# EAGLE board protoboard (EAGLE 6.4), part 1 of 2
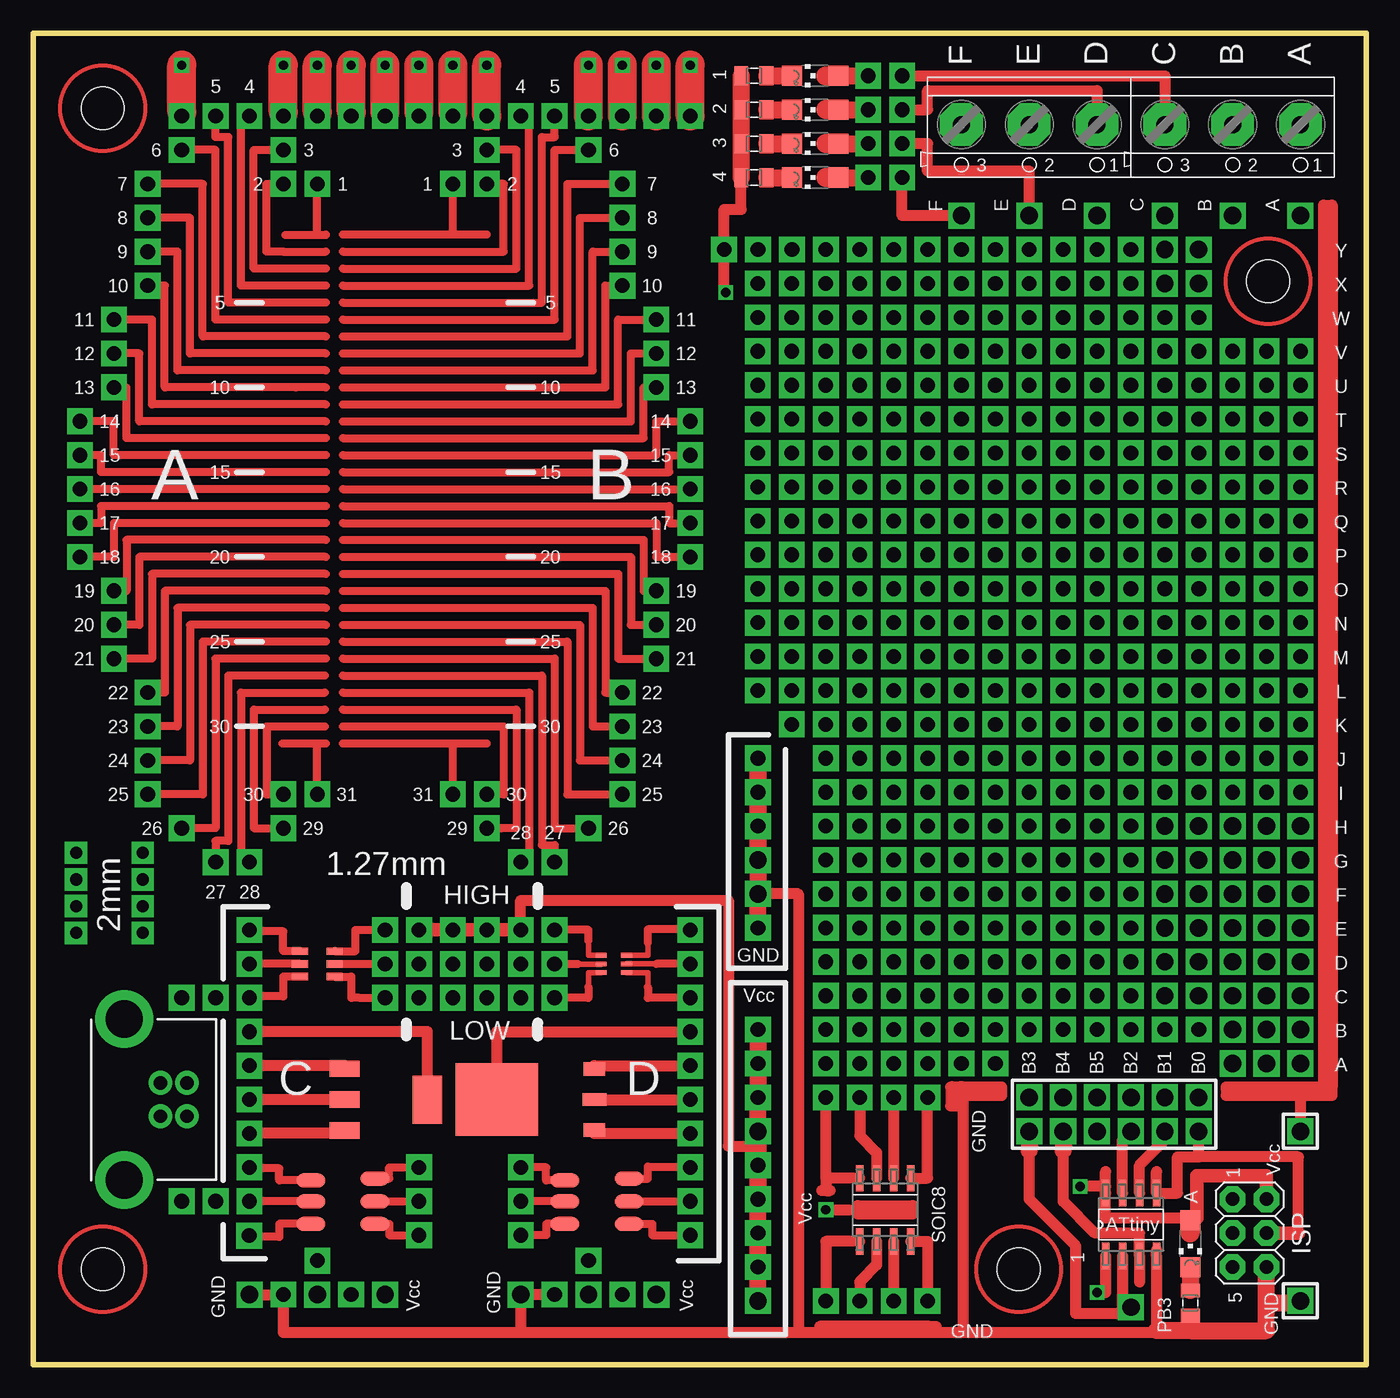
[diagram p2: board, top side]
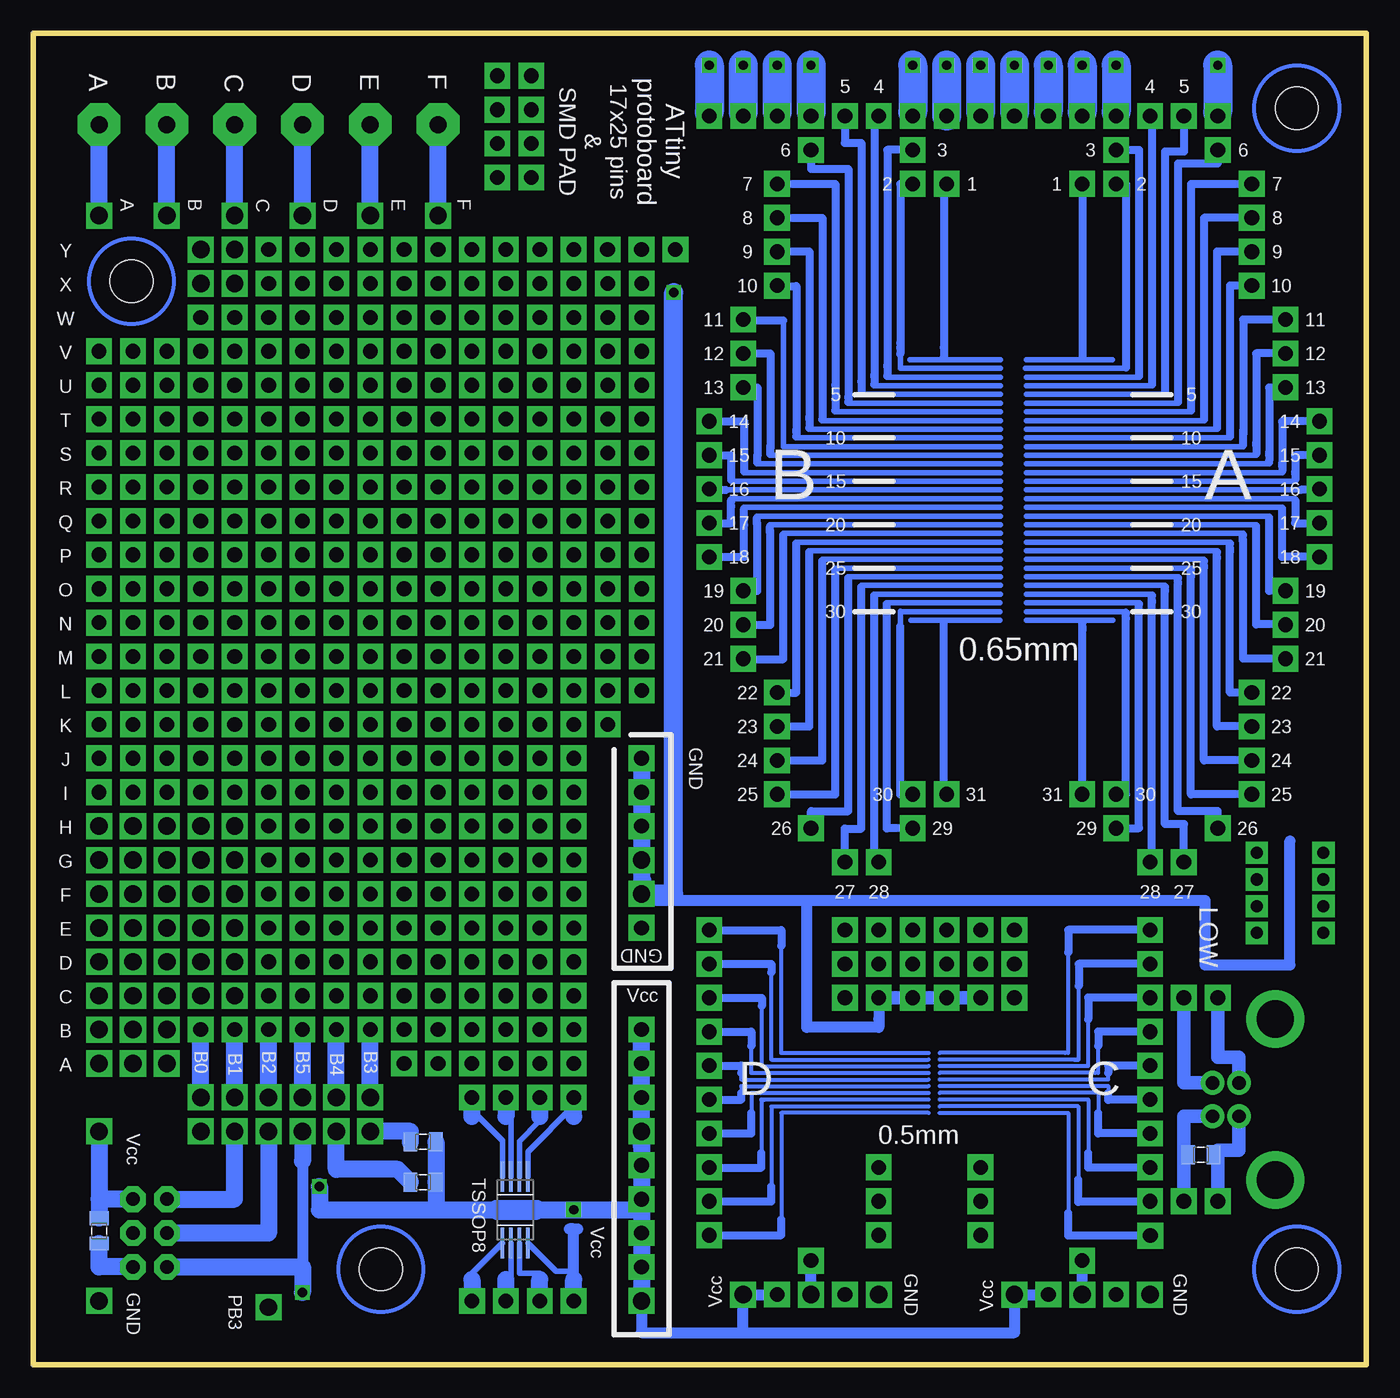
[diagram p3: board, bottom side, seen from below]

Size 99.85 x 99.7 mm. Coordinates in mm from the lower left corner, seen from the top.
Outline: 0,0 99.85,0 99.85,99.7 0,99.7 0,0
Copper layers (1*16): Top 0.035mm / dielectric 1.5mm / Bottom 0.035mm
Design rules "default *": minimum track width 10mil, minimum drill 24mil, track to track 7mil, track to pad 8mil, pad to pad 8mil, via to via 8mil, smd to smd 8mil, copper to edge 40mil, drill to drill 8mil, minimum pad ring 10mil, minimum via ring 8mil, stop-mask expansion 4mil, vias tented up to drill 0mil, thermal gap 10mil
Holes 3.2 mm at 73.82,7.14 5.19,7.14 5.19,94.08 92.51,81.12

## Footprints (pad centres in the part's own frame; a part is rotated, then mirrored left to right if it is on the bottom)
1X01 = drill 1.3 square: 1 0,0
SOIC127P600X175-8N = smd 1.981 x 0.559: 1 -2.362,1.905; 2 -2.362,0.635; 3 -2.362,-0.635; 4 -2.362,-1.905; 5 2.362,-1.905; 6 2.362,-0.635; 7 2.362,0.635; 8 2.362,1.905
0805 = smd 1.016 x 1.422: 1 -0.953,0; 2 0.953,0
TSSOP8 = smd 2.286 x 0.254: 1 -2.489,1.016; 2 -2.489,0.381; 3 -2.489,-0.254; 4 -2.489,-0.889; 5 2.489,-0.889; 6 2.489,-0.254; 7 2.489,0.381; 8 2.489,1.016
SC70-5 = smd 0.35 x 0.8: 1 -0.65,-0.95; 2 0,-0.95; 3 0.65,-0.95; 4 0.65,0.95; 5 -0.015,0.95; 6 -0.65,0.95
SOT23-5 = smd 0.55 x 1.2: 1 -0.95,-1.3; 2 0,-1.3; 3 0.95,-1.3; 4 0.95,1.3; 5 0,1.304; 6 -0.95,1.3
1X01' = drill 1.1 pad 1.93 square: 1 0,0
CZM_5/3 = drill 1.27 pad 3.2 octagon: 1 -5.08,0; 2 0,0; 3 5.08,0
CHIPLED_1206 = smd 1.5 x 1.5: A 0,-1.75; C 0,1.75
2X03 = drill 1.016 pad 1.93 octagon: 1 -2.54,-1.27; 2 -2.54,1.27; 3 0,-1.27; 4 0,1.27; 5 2.54,-1.27; 6 2.54,1.27
LED-TRICOLOR-5050-IC = smd 2.184 x 1.067: 1 -2.4,1.573; 2 -2.4,0; 3 -2.4,-1.7; 4 2.4,-1.7; 5 2.4,0; 6 2.4,1.7
SOT223 = smd 1.219 x 2.235: P-B 0,-3.099; P-C 2.311,-3.099; P_A -2.311,-3.099 | smd 3.6 x 2.2: P_POUZDRO 0,3.099
TO-252 = smd 1 x 1.6: P-A 2.28,-4.8; P-C -2.28,-4.8 | smd 0.914 x 1.778: P-B 0,-4.826 | smd 5.4 x 6.2: P_POUZDRO 0,2.5
USB-B-PTH = drill 1 pad 1.778: D+ 0,1.25; D- 1.981,1.25; GND 0,-1.25; VBUS 1.981,-1.25 | drill 2.8 pad 4.318: P$2 -2.718,6.02; SHIELD -2.718,-6.02

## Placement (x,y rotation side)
ARK-A  [1X01]  94.93,86.04 90 top
ARK-B  [1X01]  89.85,86.04 90 top
ARK-C  [1X01]  84.77,86.04 90 top
ARK-D  [1X01]  79.69,86.04 90 top
ARK-E  [1X01]  74.61,86.04 90 top
ARK-F  [1X01]  69.53,86.04 90 top
ATTINY  ATTINY__  [SOIC127P600X175-8N]  82.23,10.48 90 top
C1  [0805]  12.38,15.72 0 bottom
C8  1uF  [0805]  94.93,10 270 bottom
EMPTY1  SOIC-NIC  [SOIC127P600X175-8N]  63.82,11.59 90 top
EMPTY2  TSSOP-NIC  [TSSOP8]  63.82,11.59 270 bottom
IC1  AD8519KS  [SC70-5]  43.5,30 90 top
IC2  AD8519RJ  [SOT23-5]  21.27,30 90 top
J-A1  [1X01]  94.93,22.54 90 top
J-A2  [1X01]  92.39,22.54 90 top
J-A3  [1X01]  89.85,22.54 90 top
J-A10  [1X01']  72.07,22.54 90 top
J-A11  [1X01']  69.53,22.54 90 top
J-A12  [1X01']  66.99,22.54 90 top
J-A13  [1X01']  64.45,22.54 90 top
J-A14  [1X01']  61.91,22.54 90 top
J-A15  [1X01']  59.37,22.54 90 top
J-B1  [1X01]  94.93,25.08 90 top
J-B2  [1X01]  92.39,25.08 90 top
J-B3  [1X01]  89.85,25.08 90 top
J-B4  [1X01']  87.31,25.08 0 top
J-B5  [1X01']  84.77,25.08 0 top
J-B6  [1X01']  82.23,25.08 0 top
J-B7  [1X01']  79.69,25.08 0 top
J-B8  [1X01']  77.15,25.08 0 top
J-B9  [1X01']  74.61,25.08 0 top
J-B10  [1X01']  72.07,25.08 90 top
J-B11  [1X01']  69.53,25.08 90 top
J-B12  [1X01']  66.99,25.08 90 top
J-B13  [1X01']  64.45,25.08 90 top
J-B14  [1X01']  61.91,25.08 90 top
J-B15  [1X01']  59.37,25.08 90 top
J-C1  [1X01]  94.93,27.62 90 top
J-C2  [1X01]  92.39,27.62 90 top
J-C3  [1X01]  89.85,27.62 90 top
J-C4  [1X01]  87.31,27.62 90 top
J-C5  [1X01]  84.77,27.62 90 top
J-C6  [1X01']  82.23,27.62 90 top
J-C7  [1X01']  79.69,27.62 90 top
J-C8  [1X01']  77.15,27.62 90 top
J-C9  [1X01']  74.61,27.62 90 top
J-C10  [1X01']  72.07,27.62 90 top
J-C11  [1X01']  69.53,27.62 90 top
J-C12  [1X01']  66.99,27.62 90 top
J-C13  [1X01']  64.45,27.62 90 top
J-C14  [1X01']  61.91,27.62 90 top
J-C15  [1X01']  59.37,27.62 90 top
J-D1  [1X01]  94.93,30.16 90 top
J-D2  [1X01]  92.39,30.16 90 top
J-D3  [1X01]  89.85,30.16 90 top
J-D4  [1X01]  87.31,30.16 90 top
J-D5  [1X01]  84.77,30.16 90 top
J-D6  [1X01']  82.23,30.16 90 top
J-D7  [1X01']  79.69,30.16 90 top
J-D8  [1X01']  77.15,30.16 90 top
J-D9  [1X01']  74.61,30.16 90 top
J-D10  [1X01']  72.07,30.16 90 top
J-D11  [1X01']  69.53,30.16 90 top
J-D12  [1X01']  66.99,30.16 90 top
J-D13  [1X01']  64.45,30.16 90 top
J-D14  [1X01']  61.91,30.16 90 top
J-D15  [1X01']  59.37,30.16 90 top
J-E1  [1X01]  94.93,32.7 0 top
J-E2  [1X01]  92.39,32.7 0 top
J-E3  [1X01]  89.85,32.7 90 top
J-E4  [1X01]  87.31,32.7 90 top
J-E5  [1X01]  84.77,32.7 90 top
J-E6  [1X01']  82.23,32.7 90 top
J-E7  [1X01']  79.69,32.7 90 top
J-E8  [1X01']  77.15,32.7 90 top
J-E9  [1X01']  74.61,32.7 90 top
J-E10  [1X01']  72.07,32.7 90 top
J-E11  [1X01']  69.53,32.7 90 top
J-E12  [1X01']  66.99,32.7 0 top
J-E13  [1X01']  64.45,32.7 0 top
J-E14  [1X01']  61.91,32.7 0 top
J-E15  [1X01']  59.37,32.7 0 top
J-F1  [1X01]  94.93,35.24 0 top
J-F2  [1X01]  92.39,35.24 0 top
J-F3  [1X01]  89.85,35.24 0 top
J-F4  [1X01]  87.31,35.24 0 top
J-F5  [1X01]  84.77,35.24 0 top
J-F6  [1X01']  82.23,35.24 0 top
J-F7  [1X01']  79.69,35.24 0 top
J-F8  [1X01']  77.15,35.24 0 top
J-F9  [1X01']  74.61,35.24 0 top
J-F10  [1X01']  72.07,35.24 0 top
J-F11  [1X01']  69.53,35.24 90 top
J-F12  [1X01']  66.99,35.24 0 top
J-F13  [1X01']  64.45,35.24 0 top
J-F14  [1X01']  61.91,35.24 90 top
J-F15  [1X01']  59.37,35.24 90 top
J-G1  [1X01]  94.93,37.78 0 top
J-G2  [1X01]  92.39,37.78 0 top
J-G3  [1X01]  89.85,37.78 0 top
J-G4  [1X01]  87.31,37.78 0 top
J-G5  [1X01]  84.77,37.78 0 top
J-G6  [1X01']  82.23,37.78 0 top
J-G7  [1X01']  79.69,37.78 0 top
J-G8  [1X01']  77.15,37.78 0 top
J-G9  [1X01']  74.61,37.78 0 top
J-G10  [1X01']  72.07,37.78 0 top
J-G11  [1X01']  69.53,37.78 0 top
J-G12  [1X01']  66.99,37.78 0 top
J-G13  [1X01']  64.45,37.78 0 top
J-G14  [1X01']  61.91,37.78 0 top
J-G15  [1X01']  59.37,37.78 0 top
J-H1  [1X01]  94.93,40.32 0 top
J-H2  [1X01]  92.39,40.32 0 top
J-H3  [1X01]  89.85,40.32 0 top
J-H4  [1X01]  87.31,40.32 0 top
J-H5  [1X01]  84.77,40.32 0 top
J-H6  [1X01']  82.23,40.32 0 top
J-H7  [1X01']  79.69,40.32 0 top
J-H8  [1X01']  77.15,40.32 0 top
J-H9  [1X01']  74.61,40.32 0 top
J-H10  [1X01']  72.07,40.32 0 top
J-H11  [1X01']  69.53,40.32 0 top
J-H12  [1X01']  66.99,40.32 0 top
J-H13  [1X01']  64.45,40.32 0 top
J-H14  [1X01']  61.91,40.32 0 top
J-H15  [1X01']  59.37,40.32 0 top
J-HL-1  [1X01']  28.89,30 0 top
J-HL-2  [1X01']  31.43,30 0 top
J-HL-3  [1X01']  33.97,30 0 top
J-HL-4  [1X01']  36.51,30 0 top
J-I1  [1X01']  94.93,42.86 0 top
J-I2  [1X01']  92.39,42.86 0 top
J-I3  [1X01']  89.85,42.86 0 top
J-I4  [1X01']  87.31,42.86 0 top
J-I5  [1X01']  84.77,42.86 0 top
J-I6  [1X01']  82.23,42.86 0 top
J-I7  [1X01']  79.69,42.86 0 top
J-I8  [1X01']  77.15,42.86 0 top
J-I9  [1X01']  74.61,42.86 0 top
J-I10  [1X01']  72.07,42.86 0 top
J-I11  [1X01']  69.53,42.86 0 top
J-I12  [1X01']  66.99,42.86 0 top
J-I13  [1X01']  64.45,42.86 0 top
J-I14  [1X01']  61.91,42.86 0 top
J-I15  [1X01']  59.37,42.86 0 top
J-J1  [1X01']  94.93,45.4 0 top
J-J2  [1X01']  92.39,45.4 0 top
J-J3  [1X01']  89.85,45.4 0 top
J-J4  [1X01']  87.31,45.4 0 top
J-J5  [1X01']  84.77,45.4 0 top
J-J6  [1X01']  82.23,45.4 0 top
J-J7  [1X01']  79.69,45.4 0 top
J-J8  [1X01']  77.15,45.4 0 top
J-J9  [1X01']  74.61,45.4 0 top
J-J10  [1X01']  72.07,45.4 0 top
J-J11  [1X01']  69.53,45.4 0 top
J-J12  [1X01']  66.99,45.4 0 top
J-J13  [1X01']  64.45,45.4 0 top
J-J14  [1X01']  61.91,45.4 0 top
J-J15  [1X01']  59.37,45.4 0 top
J-K1  [1X01']  94.93,47.94 0 top
J-K2  [1X01']  92.39,47.94 0 top
J-K3  [1X01']  89.85,47.94 0 top
J-K4  [1X01']  87.31,47.94 0 top
J-K5  [1X01']  84.77,47.94 0 top
J-K6  [1X01']  82.23,47.94 0 top
J-K7  [1X01']  79.69,47.94 0 top
J-K8  [1X01']  77.15,47.94 0 top
J-K9  [1X01']  74.61,47.94 0 top
J-K10  [1X01']  72.07,47.94 0 top
J-K11  [1X01']  69.53,47.94 0 top
J-K12  [1X01']  66.99,47.94 0 top
J-K13  [1X01']  64.45,47.94 0 top
J-K14  [1X01']  61.91,47.94 0 top
J-K15  [1X01']  59.37,47.94 0 top
J-K16  [1X01']  56.82,47.94 0 top
J-L1  [1X01']  94.93,50.48 0 top
J-L2  [1X01']  92.39,50.48 0 top
J-L3  [1X01']  89.85,50.48 0 top
J-L4  [1X01']  87.31,50.48 0 top
J-L5  [1X01']  84.77,50.48 0 top
J-L6  [1X01']  82.23,50.48 0 top
J-L7  [1X01']  79.69,50.48 0 top
J-L8  [1X01']  77.15,50.48 0 top
J-L9  [1X01']  74.61,50.48 0 top
J-L10  [1X01']  72.07,50.48 0 top
J-L11  [1X01']  69.53,50.48 0 top
J-L12  [1X01']  66.99,50.48 0 top
J-L13  [1X01']  64.45,50.48 0 top
J-L14  [1X01']  61.91,50.48 0 top
J-L15  [1X01']  59.37,50.48 0 top
J-L16  [1X01']  56.82,50.48 0 top
J-L17  [1X01']  54.28,50.48 0 top
J-LED1A  [1X01']  65.09,96.52 0 top
J-LED1B  [1X01']  62.55,96.52 0 top
J-LED2A  [1X01']  65.09,93.98 0 top
J-LED2B  [1X01']  62.55,93.98 0 top
J-LED3A  [1X01']  65.09,91.44 0 top
J-LED3B  [1X01']  62.55,91.44 0 top
J-LED4A  [1X01']  65.09,88.9 0 top
J-LED4B  [1X01']  62.55,88.9 0 top
J-M1  [1X01']  94.93,53.02 0 top
J-M2  [1X01']  92.39,53.02 0 top
J-M3  [1X01']  89.85,53.02 0 top
J-M4  [1X01']  87.31,53.02 0 top
J-M5  [1X01']  84.77,53.02 0 top
J-M6  [1X01']  82.23,53.02 0 top
J-M7  [1X01']  79.69,53.02 0 top
J-M8  [1X01']  77.15,53.02 0 top
J-M9  [1X01']  74.61,53.02 0 top
J-M10  [1X01']  72.07,53.02 0 top
J-M11  [1X01']  69.53,53.02 0 top
J-M12  [1X01']  66.99,53.02 0 top
J-M13  [1X01']  64.45,53.02 0 top
J-M14  [1X01']  61.91,53.02 0 top
J-M15  [1X01']  59.37,53.02 0 top
J-M16  [1X01']  56.82,53.02 0 top
J-M17  [1X01']  54.28,53.02 0 top
J-N1  [1X01']  94.93,55.56 0 top
J-N2  [1X01']  92.39,55.56 0 top
J-N3  [1X01']  89.85,55.56 0 top
J-N4  [1X01']  87.31,55.56 0 top
J-N5  [1X01']  84.77,55.56 0 top
J-N6  [1X01']  82.23,55.56 0 top
J-N7  [1X01']  79.69,55.56 0 top
J-N8  [1X01']  77.15,55.56 0 top
J-N9  [1X01']  74.61,55.56 0 top
J-N10  [1X01']  72.07,55.56 0 top
J-N11  [1X01']  69.53,55.56 0 top
J-N12  [1X01']  66.99,55.56 0 top
J-N13  [1X01']  64.45,55.56 0 top
J-N14  [1X01']  61.91,55.56 0 top
J-N15  [1X01']  59.37,55.56 0 top
J-N16  [1X01']  56.82,55.56 0 top
J-N17  [1X01']  54.28,55.56 0 top
J-O1  [1X01']  94.93,58.1 0 top
J-O2  [1X01']  92.39,58.1 0 top
J-O3  [1X01']  89.85,58.1 0 top
J-O4  [1X01']  87.31,58.1 0 top
J-O5  [1X01']  84.77,58.1 0 top
J-O6  [1X01']  82.23,58.1 0 top
J-O7  [1X01']  79.69,58.1 0 top
J-O8  [1X01']  77.15,58.1 0 top
J-O9  [1X01']  74.61,58.1 0 top
J-O10  [1X01']  72.07,58.1 0 top
J-O11  [1X01']  69.53,58.1 0 top
J-O12  [1X01']  66.99,58.1 0 top
J-O13  [1X01']  64.45,58.1 0 top
J-O14  [1X01']  61.91,58.1 0 top
J-O15  [1X01']  59.37,58.1 0 top
J-O16  [1X01']  56.82,58.1 0 top
J-O17  [1X01']  54.28,58.1 0 top
J-P1  [1X01']  94.93,60.64 0 top
J-P2  [1X01']  92.39,60.64 0 top
J-P3  [1X01']  89.85,60.64 0 top
J-P4  [1X01']  87.31,60.64 0 top
J-P5  [1X01']  84.77,60.64 0 top
J-P6  [1X01']  82.23,60.64 0 top
J-P7  [1X01']  79.69,60.64 0 top
J-P8  [1X01']  77.15,60.64 0 top
J-P9  [1X01']  74.61,60.64 0 top
J-P10  [1X01']  72.07,60.64 0 top
J-P11  [1X01']  69.53,60.64 0 top
J-P12  [1X01']  66.99,60.64 0 top
J-P13  [1X01']  64.45,60.64 0 top
J-P14  [1X01']  61.91,60.64 0 top
J-P15  [1X01']  59.37,60.64 0 top
J-P16  [1X01']  56.82,60.64 0 top
J-P17  [1X01']  54.28,60.64 0 top
J-Q1  [1X01']  94.93,63.18 0 top
J-Q2  [1X01']  92.39,63.18 0 top
J-Q3  [1X01']  89.85,63.18 0 top
J-Q4  [1X01']  87.31,63.18 0 top
J-Q5  [1X01']  84.77,63.18 0 top
J-Q6  [1X01']  82.23,63.18 0 top
J-Q7  [1X01']  79.69,63.18 0 top
J-Q8  [1X01']  77.15,63.18 0 top
J-Q9  [1X01']  74.61,63.18 0 top
J-Q10  [1X01']  72.07,63.18 0 top
J-Q11  [1X01']  69.53,63.18 0 top
J-Q12  [1X01']  66.99,63.18 0 top
J-Q13  [1X01']  64.45,63.18 0 top
J-Q14  [1X01']  61.91,63.18 0 top
J-Q15  [1X01']  59.37,63.18 0 top
J-Q16  [1X01']  56.82,63.18 0 top
J-Q17  [1X01']  54.28,63.18 0 top
J-R1  [1X01']  94.93,65.72 0 top
J-R2  [1X01']  92.39,65.72 0 top
J-R3  [1X01']  89.85,65.72 0 top
J-R4  [1X01']  87.31,65.72 0 top
J-R5  [1X01']  84.77,65.72 0 top
J-R6  [1X01']  82.23,65.72 0 top
J-R7  [1X01']  79.69,65.72 0 top
J-R8  [1X01']  77.15,65.72 0 top
J-R9  [1X01']  74.61,65.72 0 top
J-R10  [1X01']  72.07,65.72 0 top
J-R11  [1X01']  69.53,65.72 0 top
J-R12  [1X01']  66.99,65.72 0 top
J-R13  [1X01']  64.45,65.72 0 top
J-R14  [1X01']  61.91,65.72 0 top
J-R15  [1X01']  59.37,65.72 0 top
J-R16  [1X01']  56.82,65.72 0 top
J-R17  [1X01']  54.28,65.72 0 top
J-S1  [1X01']  94.93,68.26 0 top
J-S2  [1X01']  92.39,68.26 0 top
J-S3  [1X01']  89.85,68.26 0 top
J-S4  [1X01']  87.31,68.26 0 top
J-S5  [1X01']  84.77,68.26 0 top
J-S6  [1X01']  82.23,68.26 0 top
J-S7  [1X01']  79.69,68.26 0 top
J-S8  [1X01']  77.15,68.26 0 top
J-S9  [1X01']  74.61,68.26 0 top
J-S10  [1X01']  72.07,68.26 0 top
J-S11  [1X01']  69.53,68.26 0 top
J-S12  [1X01']  66.99,68.26 0 top
J-S13  [1X01']  64.45,68.26 0 top
J-S14  [1X01']  61.91,68.26 0 top
J-S15  [1X01']  59.37,68.26 0 top
J-S16  [1X01']  56.82,68.26 0 top
J-S17  [1X01']  54.28,68.26 0 top
J-SOIC-1  [1X01']  59.37,4.76 0 top
J-SOIC-2  [1X01']  61.91,4.76 90 top
J-SOIC-3  [1X01']  64.45,4.76 90 top
J-SOIC-4  [1X01']  66.99,4.76 90 top
J-SOIC-6  [1X01']  64.45,20 0 top
J-SOIC-7  [1X01']  61.91,20 0 top
J-SOIC-8  [1X01']  59.37,20 180 top
J-T1  [1X01']  94.93,70.8 0 top
J-T2  [1X01']  92.39,70.8 0 top
J-T3  [1X01']  89.85,70.8 0 top
J-T4  [1X01']  87.31,70.8 0 top
J-T5  [1X01']  84.77,70.8 0 top
J-T6  [1X01']  82.23,70.8 0 top
J-T7  [1X01']  79.69,70.8 0 top
J-T8  [1X01']  77.15,70.8 0 top
J-T9  [1X01']  74.61,70.8 0 top
J-T10  [1X01']  72.07,70.8 0 top
J-T11  [1X01']  69.53,70.8 0 top
J-T12  [1X01']  66.99,70.8 0 top
J-T13  [1X01']  64.45,70.8 0 top
J-T14  [1X01']  61.91,70.8 0 top
J-T15  [1X01']  59.37,70.8 0 top
J-T16  [1X01']  56.82,70.8 0 top
J-T17  [1X01']  54.28,70.8 0 top
J-U1  [1X01']  94.93,73.34 0 top
J-U2  [1X01']  92.39,73.34 0 top
J-U3  [1X01']  89.85,73.34 0 top
J-U4  [1X01']  87.31,73.34 0 top
J-U5  [1X01']  84.77,73.34 0 top
J-U6  [1X01']  82.23,73.34 0 top
J-U7  [1X01']  79.69,73.34 0 top
J-U8  [1X01']  77.15,73.34 0 top
J-U9  [1X01']  74.61,73.34 0 top
J-U10  [1X01']  72.07,73.34 0 top
J-U11  [1X01']  69.53,73.34 0 top
J-U12  [1X01']  66.99,73.34 0 top
J-U13  [1X01']  64.45,73.34 0 top
J-U14  [1X01']  61.91,73.34 0 top
J-U15  [1X01']  59.37,73.34 0 top
J-U16  [1X01']  56.82,73.34 0 top
J-U17  [1X01']  54.28,73.34 0 top
J-V1  [1X01']  94.93,75.88 0 top
J-V2  [1X01']  92.39,75.88 0 top
J-V3  [1X01']  89.85,75.88 0 top
J-V4  [1X01']  87.31,75.88 0 top
J-V5  [1X01']  84.77,75.88 0 top
J-V6  [1X01']  82.23,75.88 0 top
J-V7  [1X01']  79.69,75.88 0 top
J-V8  [1X01']  77.15,75.88 0 top
J-V9  [1X01']  74.61,75.88 0 top
J-V10  [1X01']  72.07,75.88 0 top
J-V11  [1X01']  69.53,75.88 0 top
J-V12  [1X01']  66.99,75.88 0 top
J-V13  [1X01']  64.45,75.88 0 top
J-V14  [1X01']  61.91,75.88 0 top
J-V15  [1X01']  59.37,75.88 0 top
J-V16  [1X01']  56.82,75.88 0 top
J-V17  [1X01']  54.28,75.88 0 top
J-W4  [1X01']  87.31,78.42 0 top
J-W5  [1X01']  84.77,78.42 0 top
J-W6  [1X01']  82.23,78.42 0 top
J-W7  [1X01']  79.69,78.42 0 top
J-W8  [1X01']  77.15,78.42 0 top
J-W9  [1X01']  74.61,78.42 0 top
J-W10  [1X01']  72.07,78.42 0 top
J-W11  [1X01']  69.53,78.42 0 top
J-W12  [1X01']  66.99,78.42 0 top
J-W13  [1X01']  64.45,78.42 0 top
J-W14  [1X01']  61.91,78.42 0 top
J-W15  [1X01']  59.37,78.42 0 top
J-W16  [1X01']  56.82,78.42 0 top
J-W17  [1X01']  54.28,78.42 0 top
J-X4  [1X01]  87.31,80.96 0 top
J-X5  [1X01]  84.77,80.96 0 top
J-X6  [1X01']  82.23,80.96 0 top
J-X7  [1X01']  79.69,80.96 0 top
J-X8  [1X01']  77.15,80.96 0 top
J-X9  [1X01']  74.61,80.96 0 top
J-X10  [1X01']  72.07,80.96 0 top
J-X11  [1X01']  69.53,80.96 0 top
J-X12  [1X01']  66.99,80.96 0 top
J-X13  [1X01']  64.45,80.96 0 top
J-X14  [1X01']  61.91,80.96 0 top
J-X15  [1X01']  59.37,80.96 0 top
J-X16  [1X01']  56.82,80.96 0 top
J-X17  [1X01']  54.28,80.96 0 top
J-Y4  [1X01]  87.31,83.5 0 top
J-Y5  [1X01]  84.77,83.5 0 top
J-Y6  [1X01']  82.23,83.5 0 top
J-Y7  [1X01']  79.69,83.5 0 top
J-Y8  [1X01']  77.15,83.5 0 top
J-Y9  [1X01']  74.61,83.5 0 top
J-Y10  [1X01']  72.07,83.5 0 top
J-Y11  [1X01']  69.53,83.5 0 top
J-Y12  [1X01']  66.99,83.5 0 top
J-Y13  [1X01']  64.45,83.5 0 top
J-Y14  [1X01']  61.91,83.5 0 top
J-Y15  [1X01']  59.37,83.5 0 top
J-Y16  [1X01']  56.83,83.5 0 top
J-Y17  [1X01']  54.29,83.5 0 top
JP9  [1X01]  74.61,20 0 top
JP19  [1X01]  79.69,20 0 top
JP20  [1X01]  82.23,20 0 top
JP21  [1X01]  84.77,20 0 top
JP24  [1X01]  87.31,20 0 top
JP25  [1X01]  77.15,20 0 top
JP27  [1X01]  87.31,17.46 90 top
JP28  [1X01]  84.77,17.46 90 top
JP29  [1X01]  82.23,17.46 90 top
JP30  [1X01]  79.69,17.46 90 top
JP31  [1X01]  74.61,17.46 90 top
JP32  [1X01]  77.15,17.46 90 top
JP96  [1X01]  82.23,4.29 0 top
JP117  [1X01]  94.93,4.76 0 top
JP198  [1X01']  51.75,83.5 0 top
K1  CZM_5/3  [CZM_5/3]  89.85,92.87 180 top
K2  CZM_5/3  [CZM_5/3]  74.61,92.87 180 top
LED1  L-HSMS-C650  [CHIPLED_1206]  58.58,96.52 90 top
LED2  L-HSMS-C650  [CHIPLED_1206]  58.58,93.98 90 top
LED3  L-HSMS-C650  [CHIPLED_1206]  58.58,91.44 90 top
LED4  L-HSMS-C650  [CHIPLED_1206]  58.58,88.9 90 top
LED-NAP  L-HSMY-C650  [CHIPLED_1206]  86.68,9.05 180 top
P-U/PB3  [0805]  70.64,16.67 0 bottom
P-U/PB4  [0805]  70.64,13.65 0 bottom
PIN1A  [1X01']  21.27,88.42 90 top
PIN1B  [1X01']  31.43,88.42 90 top
PIN1C  [1X01']  16.19,32.54 0 top
PIN1D  [1X01']  49.21,32.54 0 top
PIN2A  [1X01']  18.73,88.42 90 top
PIN2B  [1X01']  33.97,88.42 90 top
PIN2C  [1X01']  16.19,30 90 top
PIN2D  [1X01']  49.21,30 0 top
PIN3A  [1X01']  18.73,90.96 90 top
PIN3B  [1X01']  33.97,90.96 90 top
PIN3C  [1X01']  16.19,27.46 90 top
PIN3D  [1X01']  49.21,27.46 0 top
PIN4A  [1X01']  16.19,93.5 90 top
PIN4B  [1X01']  36.51,93.5 90 top
PIN4C  [1X01']  16.19,24.92 90 top
PIN4D  [1X01']  49.21,24.92 0 top
PIN5A  [1X01']  13.65,93.5 90 top
PIN5B  [1X01']  39.05,93.5 90 top
PIN5C  [1X01']  16.19,22.38 90 top
PIN5D  [1X01']  49.21,22.38 0 top
PIN6A  [1X01']  11.11,90.96 90 top
PIN6B  [1X01']  41.59,90.96 90 top
PIN6C  [1X01']  16.19,19.84 90 top
PIN6D  [1X01']  49.21,19.84 0 top
PIN7A  [1X01']  8.57,88.42 90 top
PIN7B  [1X01']  44.13,88.42 90 top
PIN7C  [1X01']  16.19,17.3 90 top
PIN7D  [1X01']  49.21,17.3 0 top
PIN8A  [1X01']  8.57,85.88 90 top
PIN8B  [1X01']  44.13,85.88 90 top
PIN8C  [1X01']  16.19,14.76 90 top
PIN8D  [1X01']  49.21,14.76 0 top
PIN9A  [1X01']  8.57,83.34 90 top
PIN9B  [1X01']  44.13,83.34 90 top
PIN9C  [1X01']  16.19,12.22 90 top
PIN9D  [1X01']  49.21,12.22 0 top
PIN10A  [1X01']  8.57,80.8 90 top
PIN10B  [1X01']  44.13,80.8 90 top
PIN10C  [1X01']  16.16,9.65 90 top
PIN10D  [1X01']  49.21,9.68 0 top
PIN11A  [1X01']  6.03,78.26 90 top
PIN11B  [1X01']  46.67,78.26 90 top
PIN12A  [1X01']  6.03,75.72 90 top
PIN12B  [1X01']  46.67,75.72 90 top
PIN13A  [1X01']  6.03,73.18 90 top
PIN13B  [1X01']  46.67,73.18 90 top
PIN14A  [1X01']  3.49,70.64 90 top
PIN14B  [1X01']  49.21,70.64 90 top
PIN15A  [1X01']  3.49,68.1 90 top
PIN15B  [1X01']  49.21,68.1 90 top
PIN16A  [1X01']  3.49,65.56 90 top
PIN16B  [1X01']  49.21,65.56 90 top
PIN17A  [1X01']  3.49,63.02 90 top
PIN17B  [1X01']  49.21,63.02 90 top
PIN18A  [1X01']  3.49,60.48 90 top
PIN18B  [1X01']  49.21,60.48 90 top
PIN19A  [1X01']  6.03,57.94 90 top
PIN19B  [1X01']  46.67,57.94 90 top
PIN20A  [1X01']  6.03,55.4 90 top
PIN20B  [1X01']  46.67,55.4 90 top
PIN21A  [1X01']  6.03,52.86 90 top
PIN21B  [1X01']  46.67,52.86 90 top
PIN22A  [1X01']  8.57,50.32 90 top
PIN22B  [1X01']  44.13,50.32 90 top
PIN23A  [1X01']  8.57,47.78 90 top
PIN23B  [1X01']  44.13,47.78 90 top
PIN24A  [1X01']  8.57,45.24 90 top
PIN24B  [1X01']  44.13,45.24 90 top
PIN25A  [1X01']  8.57,42.7 90 top
PIN25B  [1X01']  44.13,42.7 90 top
PIN26A  [1X01']  11.11,40.16 90 top
PIN26B  [1X01']  41.59,40.16 90 top
PIN27A  [1X01']  13.65,37.62 90 top
PIN27B  [1X01']  39.05,37.62 90 top
PIN28A  [1X01']  16.19,37.62 90 top
PIN28B  [1X01']  36.51,37.62 90 top
PIN29A  [1X01']  18.73,40.16 90 top
PIN29B  [1X01']  33.97,40.16 90 top
PIN30A  [1X01']  18.73,42.7 90 top
PIN30B  [1X01']  33.97,42.7 90 top
PIN31A  [1X01']  21.27,42.7 90 top
PIN31B  [1X01']  31.43,42.7 90 top
PIN-BOK1  [1X01']  11.11,93.5 0 top
PIN-BOK2  [1X01']  18.73,93.5 0 top
PIN-BOK3  [1X01']  21.27,93.5 0 top
PIN-BOK4  [1X01']  23.81,93.5 0 top
PIN-BOK5  [1X01']  26.35,93.5 0 top
PIN-BOK6  [1X01']  28.89,93.5 0 top
PIN-BOK7  [1X01']  31.43,93.5 0 top
PIN-BOK8  [1X01']  33.97,93.5 0 top
PIN-BOK9  [1X01']  41.59,93.5 0 top
PIN-BOK10  [1X01']  44.13,93.5 0 top
PIN-BOK11  [1X01']  46.67,93.5 0 top
PIN-BOK12  [1X01']  49.21,93.5 0 top
PIN-SOT1  [1X01']  26.35,32.54 0 top
PIN-SOT2  [1X01']  26.35,30 0 top
PIN-SOT3  [1X01']  26.35,27.46 0 top
PIN-SOT4  [1X01']  28.89,14.76 0 top
PIN-SOT5  [1X01']  28.89,12.22 0 top
PIN-SOT6  [1X01']  28.89,9.68 0 top
PIN-SOT7  [1X01']  39.05,32.54 0 top
PIN-SOT8  [1X01']  39.05,30 0 top
PIN-SOT9  [1X01']  39.05,27.46 0 top
PIN-SOT10  [1X01']  36.51,14.76 0 top
PIN-SOT11  [1X01']  36.51,12.22 0 top
PIN-SOT12  [1X01']  36.51,9.68 0 top
PINGND-1  [1X01']  28.89,27.46 0 top
PINGND-2  [1X01']  31.43,27.46 0 top
PINGND-3  [1X01']  33.97,27.46 0 top
PINGND-4  [1X01']  36.51,27.46 0 top
PINGND-5  [1X01]  16.19,5.24 90 top
PINGND-6  [1X01']  18.73,5.24 0 top
PINGND-7  [1X01]  36.51,5.24 90 top
PINGND-8  [1X01']  39.05,5.24 0 top
PINGND-9  [1X01']  54.29,32.7 90 top
PINGND-10  [1X01]  54.29,35.24 90 top
PINGND-11  [1X01]  54.29,37.78 90 top
PINGND-12  [1X01']  54.29,40.32 90 top
PINGND-13  [1X01']  54.29,42.86 90 top
PINGND-14  [1X01']  54.29,45.4 90 top
PINPOT1A  [1X01']  21.27,7.78 0 top
PINPOT1B  [1X01]  21.27,5.24 90 top
PINPOT2A  [1X01']  41.59,7.78 0 top
PINPOT2B  [1X01]  41.59,5.24 90 top
PINUSB1  [1X01']  13.65,12.23 0 top
PINUSB2  [1X01']  13.65,27.47 0 top
PINUSB3  [1X01']  11.11,27.47 0 top
PINUSB4  [1X01']  11.11,12.23 0 top
PINVCC-1  [1X01']  28.89,32.54 0 top
PINVCC-2  [1X01']  31.43,32.54 0 top
PINVCC-3  [1X01']  33.97,32.54 90 top
PINVCC-4  [1X01']  36.51,32.54 90 top
PINVCC-5  [1X01]  26.35,5.24 90 top
PINVCC-6  [1X01']  23.81,5.24 0 top
PINVCC-7  [1X01]  46.67,5.24 90 top
PINVCC-8  [1X01']  44.13,5.24 0 top
PINVCC-9  [1X01']  54.29,25.08 0 top
PINVCC-10  [1X01']  54.29,22.54 0 top
PINVCC-11  [1X01']  54.29,20 0 top
PINVCC-12  [1X01]  54.29,17.46 90 top
PINVCC-13  [1X01']  54.29,14.92 180 top
PINVCC-14  [1X01']  54.29,12.38 90 top
PINVCC-15  [1X01']  54.29,9.84 90 top
PINVCC-16  [1X01']  54.29,7.3 90 top
PINVCC-17  [1X01]  54.29,4.76 90 top
PINVCC-18  [1X01]  94.93,17.46 0 top
RLED1  [0805]  53.98,96.52 0 top
RLED2  [0805]  53.98,93.98 0 top
RLED3  [0805]  53.98,91.44 0 top
RLED4  [0805]  53.98,88.9 0 top
RLED-NAP  [0805]  86.68,4.6 90 top
SOIC-5  [1X01']  66.99,20 0 top
TINY-ISP  [2X03]  91.12,9.84 270 top
U1  WS2812  [LED-TRICOLOR-5050-IC]  23.18,12.22 0 top
U2  WS2812  [LED-TRICOLOR-5050-IC]  42.23,12.22 0 top
U6  [SOT223]  26.43,19.84 270 top
U7  +12v  [TO-252]  37.22,19.84 90 top
X1  USBPTH  [USB-B-PTH]  9.53,19.84 0 top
